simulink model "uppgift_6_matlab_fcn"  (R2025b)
settings: Solver=VariableStepAuto  StartTime=0.0  StopTime=10.0  RelTol=1e-3
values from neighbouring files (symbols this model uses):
  AFs = 14.6    [Lektion_2.m]
  Ki = 0.1    [Lektion_2.m]
  Kp = 0    [Lektion_2.m]

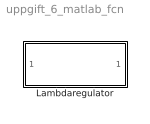
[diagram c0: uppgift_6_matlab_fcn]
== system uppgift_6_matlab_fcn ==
  Lambdaregulator : Subsystem

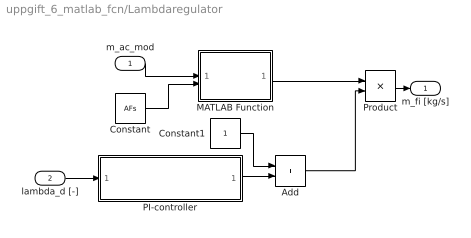
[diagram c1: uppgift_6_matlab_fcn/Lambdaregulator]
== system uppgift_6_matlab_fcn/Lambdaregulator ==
  m_ac_mod : Inport
  lambda_d [-] : Inport  Port=2
  Add : Sum
  Constant : Constant  Value=AFs
  Constant1 : Constant
  MATLAB Function : MATLAB Function  TreatAsAtomicUnit=on
  PI-controller : Subsystem
  Product : Product
  m_fi [kg/s] : Outport
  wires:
  m_ac_mod/1 -> MATLAB Function/1(m_ac)
  Constant/1 -> MATLAB Function/2(AFs)
  Constant1/1 -> Add/1
  Add/1 -> Product/2
  Product/1 -> m_fi [kg/s]/1
  PI-controller/1("Lambda_controlled ") -> Add/2
  lambda_d [-]/1 -> PI-controller/1(lambda_d)
  MATLAB Function/1(m_fi) -> Product/1

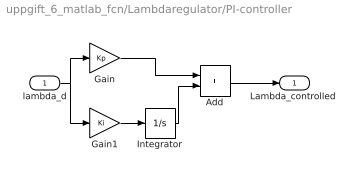
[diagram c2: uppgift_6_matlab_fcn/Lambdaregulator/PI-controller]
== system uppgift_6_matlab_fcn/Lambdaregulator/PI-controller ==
  lambda_d : Inport
  Add : Sum
  Gain : Gain  Gain=Kp
  Gain1 : Gain  Gain=Ki
  Integrator : Integrator
  "Lambda_controlled " : Outport
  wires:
  Add/1 -> "Lambda_controlled "/1
  Gain1/1 -> Integrator/1
  Integrator/1 -> Add/2
  lambda_d/1 -> Gain/1, Gain1/1
  Gain/1 -> Add/1

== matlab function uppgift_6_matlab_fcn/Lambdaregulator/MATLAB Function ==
function m_fi = fcn(m_ac, AFs)

m_fi = m_ac/AFs;
